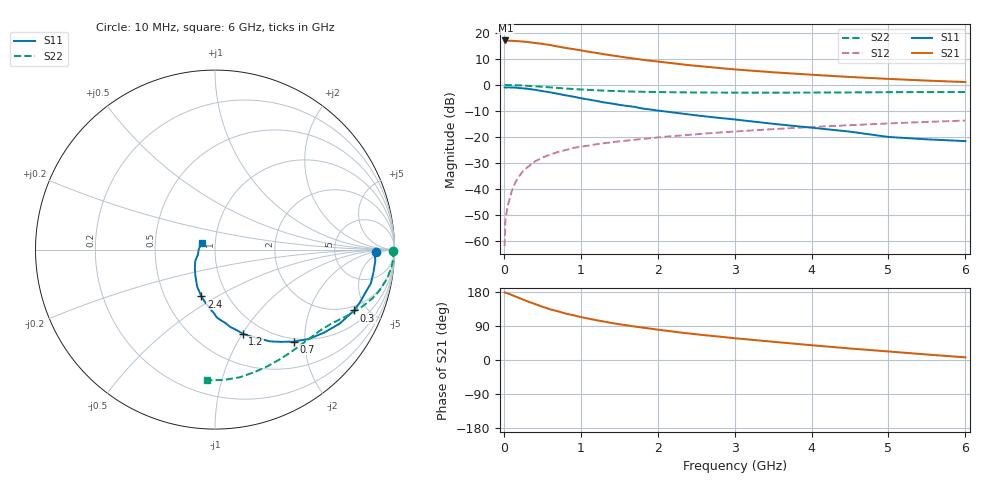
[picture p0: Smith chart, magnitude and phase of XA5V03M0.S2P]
! SIEMENS Discrete & RF Semiconductors
! BFY180
! Si NPN RF Bipolar Junction Transistor in MICRO-X
! VCE = 5 V  IC = 3 mA
! Common Emitter S-Parameters:  May  1997
# GHz  S  MA  R  50
!  f  S11  S21  S12  S22
! GHz  MAG  ANG  MAG  ANG  MAG  ANG  MAG  ANG
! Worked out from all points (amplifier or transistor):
!   36 points, 10 MHz to 6 GHz, reference 50 ohm
!   highest |S21| = 17.1 dB at 20 MHz (marker M1)
!   |S21| within 3 dB of that: start of sweep to 830.4 MHz
!   unconditionally stable (mu >= 1): 2.42 GHz to end of sweep
!   at 250 MHz: K = 0.15, MSG = 24.9 dB, |S12| = -33.1 dB
!   at 1.4 GHz: K = 0.77, MSG = 16.7 dB, |S12| = -22.0 dB
!   at 6 GHz: K = 1.06, MAG = 5.9 dB, |S12| = -13.7 dB
!   S11 on the Smith chart (normalised r, x): 10 MHz: 18, -2; 300 MHz: 1.72, -4.10; 700 MHz: 0.95, -1.78; 1.2 GHz: 0.81, -1.00; 2.4 GHz: 0.76, -0.43; 6 GHz: 0.86, +0.07
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0.01  0.8952 -0.7  7.104 178.5  0.0008 82.4  0.9934 -0.3
0.02  0.8888 -1.5  7.14 177.6  0.0025 86.4  0.9999 -0.8
0.05  0.8955 -3.9  7.021 175.8  0.0047 85.7  0.9943 -1.9
0.1  0.8918 -8.2  7.049 171.8  0.0088 87.1  0.9924 -3.8
0.15  0.8888 -12.2  6.972 167.6  0.0135 82.9  0.9885 -5.7
0.3  0.8463 -23.6  6.699 155.4  0.0257 76.3  0.9627 -10.9
0.5  0.7622 -37.5  6.148 140.6  0.0401 68.2  0.9207 -16.9
0.6  0.7205 -43.8  5.833 133.8  0.0458 65.2  0.8966 -19.4
0.7  0.6755 -49.3  5.471 128.7  0.0513 62.2  0.8751 -21.6
0.8  0.633 -54.3  5.133 122.8  0.056 60.4  0.8534 -23.6
1  0.5563 -63.3  4.608 113.4  0.065 56.2  0.8183 -27.1
1.1  0.5233 -67.6  4.338 109.2  0.0684 54.7  0.8028 -28.5
1.2  0.4937 -71.7  4.117 105.1  0.0725 53.5  0.7896 -30.0
1.4  0.4395 -78.8  3.69 97.7  0.079 51.4  0.7666 -32.7
1.7  0.3786 -88.4  3.199 88.4  0.0885 49.1  0.7431 -36.7
2.2  0.2963 -101.0  2.601 75.0  0.1043 45.4  0.7235 -43.1
2.4  0.2716 -106.3  2.399 70.1  0.1097 44.3  0.7176 -45.5
3  0.2172 -118.0  1.985 57.5  0.1273 40.5  0.711 -53.0
3.5  0.179 -127.8  1.749 48.1  0.1415 37.4  0.7099 -59.3
4.5  0.1266 -150.3  1.42 30.4  0.1687 30.2  0.7174 -72.3
5.5  0.0901 178.1  1.21 14.5  0.1949 22.6  0.728 -86.3
6  0.0834 152.7  1.134 7.0  0.2067 18.4  0.7289 -93.4
